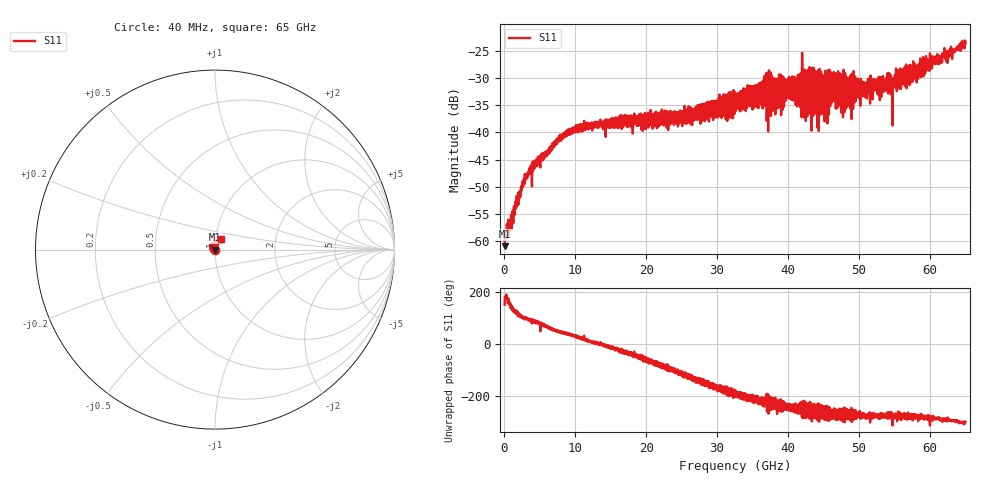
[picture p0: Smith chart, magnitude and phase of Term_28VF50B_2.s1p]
! Created Tue Jul 15 17:40:31 2008
# hz S ma R 50
! 2 Port Network Data from blockName block
! freq  magS11  angS11
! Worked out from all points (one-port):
!   1601 points, 40 MHz to 65 GHz, reference 50 ohm
!   lowest |S11| = -60.9 dB at 40 MHz (marker M1), VSWR 1.00, Z = 49.9 + j0.0463 ohm
!   |S11| at or under -10 dB: start of sweep to end of sweep
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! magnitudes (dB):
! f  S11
! 40 MHz  -60.9
! 3.207 GHz  -48.4
! 8.16 GHz  -40.7
! 11.41 GHz  -39.6
! 16.28 GHz  -37.3
! 24.4 GHz  -36.3
! 32.52 GHz  -32.6
! 36.62 GHz  -35.1
! 37.31 GHz  -28.6
! 37.59 GHz  -37.0
! 37.92 GHz  -30.0
! 40.64 GHz  -33.5
! 41.61 GHz  -29.5
! 42.1 GHz  -28.6
! 42.63 GHz  -28.8
! 42.91 GHz  -36.5
! 43.64 GHz  -28.2
! 43.73 GHz  -36.6
! 44.05 GHz  -29.0
! 44.54 GHz  -36.8
! 45.23 GHz  -28.7
! 46.32 GHz  -34.1
! 48.76 GHz  -35.6
! 51.64 GHz  -29.6
! 54.12 GHz  -32.9
! 54.65 GHz  -30.0
! 56.88 GHz  -29.8
! 65 GHz  -23.6
